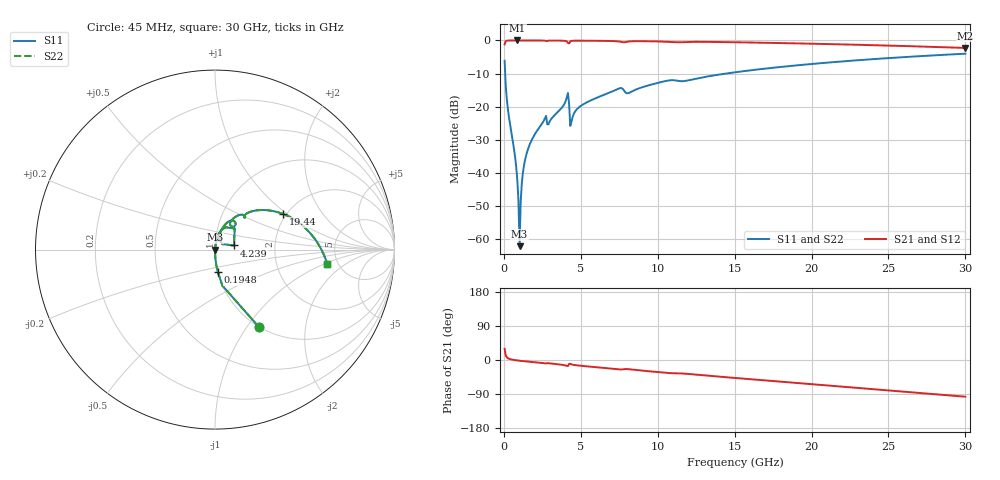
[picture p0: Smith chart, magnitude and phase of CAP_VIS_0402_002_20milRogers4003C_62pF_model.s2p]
! S-parameter model data by Modelithics Inc.  support@modelithics.com  813-866-6335  Tampa FL USA
! S-Parameter data specifications:
! Substrate: 20-mil Rogers 4003C, substrate thickness, H=0.508mm, Dielectric constant, Er=3.75
! PCB Mounting Pad Footprint: Pad width, PadW=0.50mm , Pad length, PadL=0.50mm , Pad gap, PadG (edge-to-edge)=0.40mm , Reference planes=1.4mm apart
! Created Wed Nov 18 12:56:17 2015
# hz S ma R 50
! 2 Port Network Data from SP1.SP block
! freq  magS11  angS11  magS21  angS21  magS12  angS12  magS22  angS22
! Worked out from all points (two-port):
!   401 points, 45 MHz to 30 GHz, reference 50 ohm
!   highest |S21| = -0.01 dB at 868.8 MHz (marker M1); lowest = -2.3 dB at 30 GHz (marker M2)
!   |S21| within 3 dB of the highest: start of sweep to end of sweep
!   lowest |S11| = -62.2 dB at 1.019 GHz (marker M3), VSWR 1.00, Z = 50.1 + j0.0104 ohm
!   |S11| at or under -10 dB: 83.12 MHz to 14.45 GHz (14.37 GHz wide, 198 % of centre)
!   |S22| runs from -62.2 to -4.0 dB; largest |S21 - S12| = 0
!   S11 on the Smith chart (normalised r, x): 45 MHz: 1.00, -1.13; 194.8 MHz: 1.00, -0.25; 4.239 GHz: 1.24, +0.06; 19.44 GHz: 1.93, +0.94; 30 GHz: 4.11, -1.09
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4.5e7  0.4934 -60.5  0.8696 29.5  0.8696 29.5  0.4934 -60.5
1.94775e8  0.1255 -83.0  0.9917 6.8  0.9917 6.8  0.1255 -83.0
7.189875e8  0.01781 -88.2  0.9992 -0.3  0.9992 -0.3  0.01781 -88.2
8.687625e8  0.007973 -86.0  0.9992 -1.2  0.9992 -1.2  0.007973 -86.0
1.018538e9  0.0007791 7.7  0.9992 -1.9  0.9992 -1.9  0.0007791 7.7
1.168312e9  0.007159 80.8  0.9991 -2.6  0.9991 -2.6  0.007159 80.8
1.2432e9  0.01036 82.4  0.9991 -2.9  0.9991 -2.9  0.01036 82.4
1.392975e9  0.01636 83.3  0.9989 -3.5  0.9989 -3.5  0.01636 83.3
1.917188e9  0.03509 82.6  0.9982 -5.6  0.9982 -5.6  0.03509 82.6
2.591175e9  0.0611 78.9  0.9951 -8.3  0.9951 -8.3  0.0611 78.9
4.014038e9  0.1213 70.1  0.981 -14.4  0.981 -14.4  0.1213 70.1
4.2387e9  0.1083 12.3  0.8991 -10.3  0.8991 -10.3  0.1083 12.3
4.463362e9  0.06944 70.2  0.9884 -12.3  0.9884 -12.3  0.06944 70.2
5.062462e9  0.105 73.1  0.9917 -15.5  0.9917 -15.5  0.105 73.1
7.458862e9  0.1876 60.0  0.9647 -24.7  0.9647 -24.7  0.1876 60.0
8.057962e9  0.1591 56.2  0.9606 -24.1  0.9606 -24.1  0.1591 56.2
1.007992e10  0.2307 55.8  0.9645 -32.2  0.9645 -32.2  0.2307 55.8
1.50225e10  0.33 41.8  0.9387 -47.4  0.9387 -47.4  0.33 41.8
1.944086e10  0.4288 27.5  0.8987 -62.0  0.8987 -62.0  0.4288 27.5
2.003996e10  0.4415 25.6  0.8926 -63.9  0.8926 -63.9  0.4415 25.6
2.505742e10  0.542 9.1  0.8353 -80.4  0.8353 -80.4  0.542 9.1
3e10  0.6305 -7.3  0.7705 -96.9  0.7705 -96.9  0.6305 -7.3
